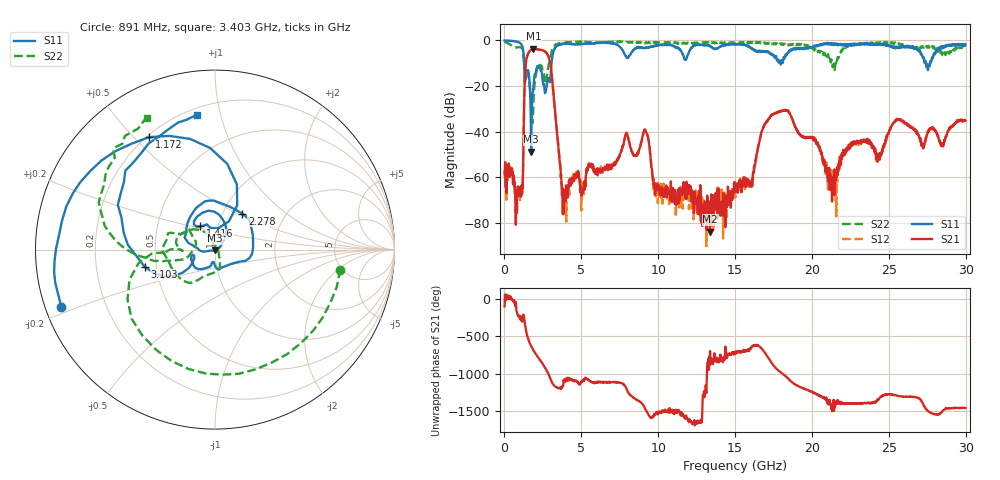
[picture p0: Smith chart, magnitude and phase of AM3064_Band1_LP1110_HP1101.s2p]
# Hz S DB R 50.0
!freq dBS11 angS11 dBS21 angS21 dBS12 angS12 dBS22 angS22
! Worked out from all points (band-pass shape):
!   1600 points, 10 MHz to 29.98 GHz, reference 50 ohm
!   highest |S21| = -3.70 dB at 1.884 GHz (marker M1); lowest = -83.8 dB at 13.37 GHz (marker M2)
!   |S21| within 3 dB of the highest: 1.488 GHz to 2.838 GHz (1.35 GHz wide, 62.4 % of centre)
!   lowest |S11| = -48.8 dB at 1.734 GHz (marker M3), VSWR 1.01, Z = 50.1 - j0.344 ohm
!   |S11| at or under -10 dB: 1.277 GHz to 3.064 GHz (1.787 GHz wide, 82.3 % of centre); 17.94465 GHz to 17.99381 GHz (49.16 MHz wide, 0.274 % of centre); 27.4 GHz to 27.68 GHz (282.1 MHz wide, 1.02 % of centre)
!   |S22| runs from -36.3 to -0.4 dB; largest |S21 - S12| = 0.01
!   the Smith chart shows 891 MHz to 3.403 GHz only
!   S11 on the Smith chart (normalised r, x): 891 MHz: 0.05, -0.18; 1.172 GHz: 0.21, +0.55; 1.416 GHz: 0.82, +0.22; 2.278 GHz: 1.23, +0.53; 3.103 GHz: 0.43, -0.10; 3.403 GHz: 0.24, +0.85
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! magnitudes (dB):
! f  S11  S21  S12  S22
! 10 MHz  0.0  -58.1  -56.8  -0.4
! 891 MHz  -0.8  -65.1  -66.8  -3.0
! 1.172 GHz  -2.8  -64.9  -66.7  -4.1
! 1.416 GHz  -16.3  -8.8  -8.7  -14.9
! 1.734 GHz  -48.8  -4.1  -4.0  -25.1
! 1.884 GHz  -20.4  -3.7  -3.7  -27.7
! 2.278 GHz  -12.0  -4.1  -4.1  -10.9
! 3.103 GHz  -7.9  -16.9  -17.1  -4.0
! 3.403 GHz  -2.4  -39.1  -39.0  -1.6
! 3.871 GHz  -1.4  -68.8  -71.9  -1.1
! 5.015 GHz  -1.6  -68.0  -64.4  -0.6
! 9.157 GHz  -3.4  -39.3  -39.1  -1.1
! 10 GHz  -2.2  -64.5  -62.5  -0.9
! 13.37 GHz  -2.5  -83.8  -76.8  -0.9
! 15 GHz  -1.8  -63.9  -67.7  -1.2
! 16.02 GHz  -3.2  -64.2  -62.1  -0.8
! 17.46 GHz  -6.6  -32.4  -32.5  -1.3
! 19.99 GHz  -3.2  -42.5  -42.5  -3.0
! 21.3 GHz  -1.7  -70.6  -59.4  -9.1
! 22.43 GHz  -1.9  -45.7  -46.5  -2.7
! 25 GHz  -2.0  -40.8  -39.9  -1.2
! 29.98 GHz  -1.7  -35.2  -34.9  -2.9
